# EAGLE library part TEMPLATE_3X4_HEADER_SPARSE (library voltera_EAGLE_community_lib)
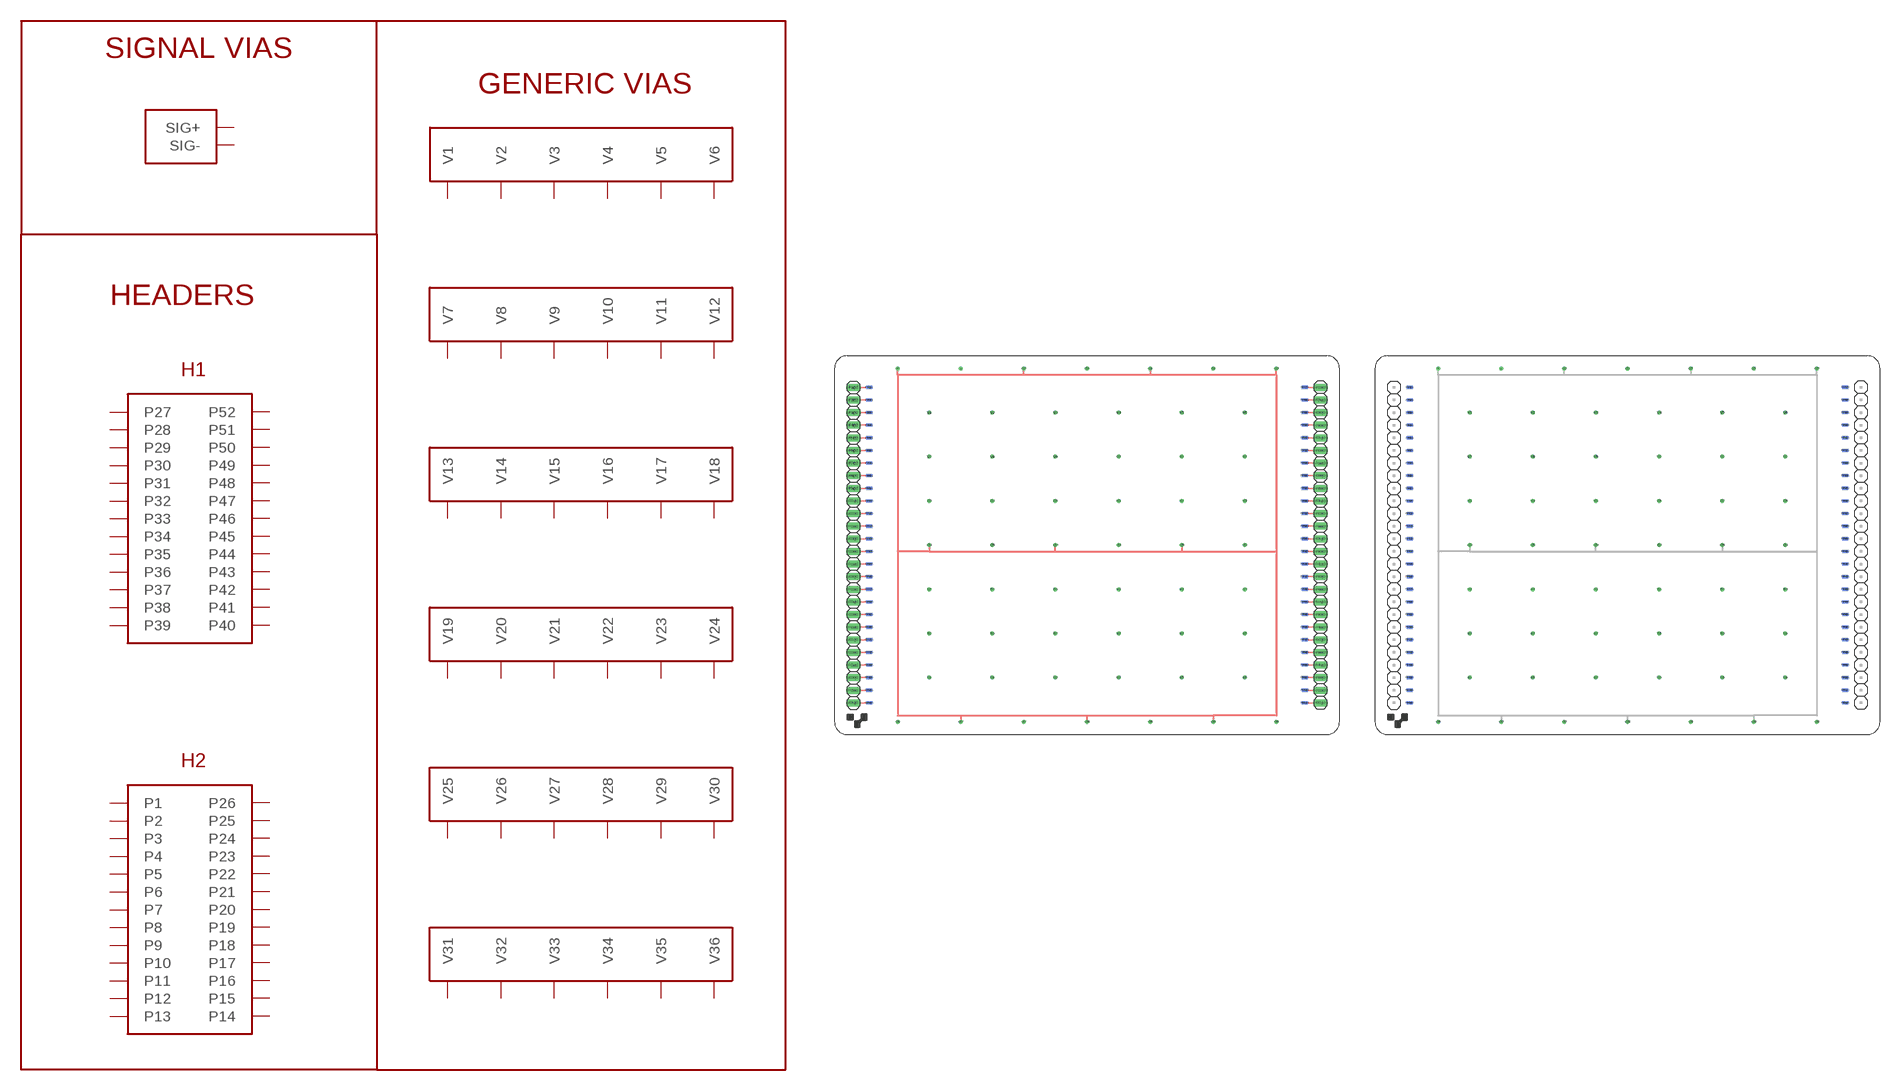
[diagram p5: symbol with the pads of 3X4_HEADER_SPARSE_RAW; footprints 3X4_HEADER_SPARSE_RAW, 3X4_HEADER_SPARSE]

Designator prefix -

## TEMPLATE_3X4_HEADER_SPARSE_RAW  [3X4_HEADER_SPARSE_RAW]
+  SIG+
+@1  SIG+
+@2  SIG+
+@3  SIG+
+@4  SIG+
+@5  SIG+
+@6  SIG+
+@7  SIG+
+@8  SIG+
+@9  SIG+
-  SIG-
-@1  SIG-
-@2  SIG-
-@3  SIG-
-@4  SIG-
-@5  SIG-
-@6  SIG-
-@7  SIG-
-@8  SIG-
-@9  SIG-
P1  P1
P1@1  P1
P1@2  P1
P2  P2
P2@1  P2
P2@2  P2
P3  P3
P3@1  P3
P3@2  P3
P4  P4
P4@1  P4
P4@2  P4
P5  P5
P5@1  P5
P5@2  P5
P6  P6
P6@1  P6
P6@2  P6
P7  P7
P7@1  P7
P7@2  P7
P8  P8
P8@1  P8
P8@2  P8
P9  P9
P9@1  P9
P9@2  P9
P10  P10
P10@1  P10
P10@2  P10
P11  P11
P11@1  P11
P11@2  P11
P12  P12
P12@1  P12
P12@2  P12
P13  P13
P13@1  P13
P13@2  P13
P14  P14
P14@1  P14
P14@2  P14
P15  P15
P15@1  P15
P15@2  P15
P16  P16
P16@1  P16
P16@2  P16
P17  P17
P17@1  P17
P17@2  P17
P18  P18
P18@1  P18
P18@2  P18
P19  P19
P19@1  P19
P19@2  P19
P20  P20
P20@1  P20
P20@2  P20
P21  P21
P21@1  P21
P21@2  P21
P22  P22
P22@1  P22
P22@2  P22
P23  P23
P23@1  P23
P23@2  P23
P24  P24
P24@1  P24
P24@2  P24
P25  P25
P25@1  P25
P25@2  P25
P26  P26
P26@1  P26
P26@2  P26
P27  P27
P27@1  P27
P27@2  P27
P28  P28
P28@1  P28
P28@2  P28
P29  P29
P29@1  P29
P29@2  P29
P30  P30
P30@1  P30
P30@2  P30
P31  P31
P31@1  P31
P31@2  P31
P32  P32
P32@1  P32
P32@2  P32
P33  P33
P33@1  P33
P33@2  P33
P34  P34
P34@1  P34
P34@2  P34
P35  P35
P35@1  P35
P35@2  P35
P36  P36
P36@1  P36
P36@2  P36
P37  P37
P37@1  P37
P37@2  P37
P38  P38
P38@1  P38
P38@2  P38
P39  P39
P39@1  P39
P39@2  P39
P40  P40
P40@1  P40
P40@2  P40
P41  P41
P41@1  P41
P41@2  P41
P42  P42
P42@1  P42
P42@2  P42
P43  P43
P43@1  P43
P43@2  P43
P44  P44
P44@1  P44
P44@2  P44
P45  P45
P45@1  P45
P45@2  P45
P46  P46
P46@1  P46
P46@2  P46
P47  P47
P47@1  P47
P47@2  P47
P48  P48
P48@1  P48
P48@2  P48
P49  P49
P49@1  P49
P49@2  P49
P50  P50
P50@1  P50
P50@2  P50
P51  P51
P51@1  P51
P51@2  P51
P52  P52
P52@1  P52
P52@2  P52
V1  V1
V2  V2
V3  V3
V4  V4
V5  V5
V6  V6
V7  V7
V8  V8
V9  V9
V10  V10
V11  V11
V12  V12
V13  V13
V14  V14
V15  V15
V16  V16
V17  V17
V18  V18
V19  V19
V20  V20
V21  V21
V22  V22
V23  V23
V24  V24
V25  V25
V26  V26
V27  V27
V28  V28
V29  V29
V30  V30
V31  V31
V32  V32
V33  V33
V34  V34
V35  V35
V36  V36

## TEMPLATE_3X4_HEADER_SPARSE_TEMPLATE  [3X4_HEADER_SPARSE]
+  SIG+
+@1  SIG+
+@2  SIG+
+@3  SIG+
+@4  SIG+
+@5  SIG+
+@6  SIG+
+@7  SIG+
+@8  SIG+
+@9  SIG+
-  SIG-
-@1  SIG-
-@2  SIG-
-@3  SIG-
-@4  SIG-
-@5  SIG-
-@6  SIG-
-@7  SIG-
-@8  SIG-
-@9  SIG-
P1  P1
P1@1  P1
P2  P2
P2@1  P2
P3  P3
P3@1  P3
P4  P4
P4@1  P4
P5  P5
P5@1  P5
P6  P6
P6@1  P6
P7  P7
P7@1  P7
P8  P8
P8@1  P8
P9  P9
P9@1  P9
P10  P10
P10@1  P10
P11  P11
P11@1  P11
P12  P12
P12@1  P12
P13  P13
P13@1  P13
P14  P14
P14@1  P14
P15  P15
P15@1  P15
P16  P16
P16@1  P16
P17  P17
P17@1  P17
P18  P18
P18@1  P18
P19  P19
P19@1  P19
P20  P20
P20@1  P20
P21  P21
P21@1  P21
P22  P22
P22@1  P22
P23  P23
P23@1  P23
P24  P24
P24@1  P24
P25  P25
P25@1  P25
P26  P26
P26@1  P26
P27  P27
P27@1  P27
P28  P28
P28@1  P28
P29  P29
P29@1  P29
P30  P30
P30@1  P30
P31  P31
P31@1  P31
P32  P32
P32@1  P32
P33  P33
P33@1  P33
P34  P34
P34@1  P34
P35  P35
P35@1  P35
P36  P36
P36@1  P36
P37  P37
P37@1  P37
P38  P38
P38@1  P38
P39  P39
P39@1  P39
P40  P40
P40@1  P40
P41  P41
P41@1  P41
P42  P42
P42@1  P42
P43  P43
P43@1  P43
P44  P44
P44@1  P44
P45  P45
P45@1  P45
P46  P46
P46@1  P46
P47  P47
P47@1  P47
P48  P48
P48@1  P48
P49  P49
P49@1  P49
P50  P50
P50@1  P50
P51  P51
P51@1  P51
P52  P52
P52@1  P52
V1  V1
V2  V2
V3  V3
V4  V4
V5  V5
V6  V6
V7  V7
V8  V8
V9  V9
V10  V10
V11  V11
V12  V12
V13  V13
V14  V14
V15  V15
V16  V16
V17  V17
V18  V18
V19  V19
V20  V20
V21  V21
V22  V22
V23  V23
V24  V24
V25  V25
V26  V26
V27  V27
V28  V28
V29  V29
V30  V30
V31  V31
V32  V32
V33  V33
V34  V34
V35  V35
V36  V36

## Footprint 3X4_HEADER_SPARSE_RAW (pad centres in mm)
drill 0.3 pad 0.8: + 12.7,73.66; +@1 38.1,73.66; +@2 63.5,73.66; +@3 19.05,38.1; +@4 44.45,38.1; +@5 69.85,38.1; +@6 88.9,73.66; +@7 25.4,2.54; +@8 50.8,2.54; +@9 76.2,2.54; - 25.4,73.66; -@1 50.8,73.66; -@2 76.2,73.66; -@3 82.55,38.1; -@4 57.15,38.1; -@5 31.75,38.1; -@6 12.7,2.54; -@7 38.1,2.54; -@8 63.5,2.54; -@9 88.9,2.54; V1 19.05,64.77; V2 31.75,64.77; V3 44.45,64.77; V4 57.15,64.77; V5 69.85,64.77; V6 82.55,64.77; V7 19.05,55.88; V8 31.75,55.88; V9 44.45,55.88; V10 57.15,55.88; V11 69.85,55.88; V12 82.55,55.88; V13 19.05,46.99; V14 31.75,46.99; V15 44.45,46.99; V16 57.15,46.99; V17 69.85,46.99; V18 82.55,46.99; V19 19.05,29.21; V20 31.75,29.21; V21 44.45,29.21; V22 57.15,29.21; V23 69.85,29.21; V24 82.55,29.21; V25 19.05,20.32; V26 31.75,20.32; V27 44.45,20.32; V28 57.15,20.32; V29 69.85,20.32; V30 82.55,20.32; V31 19.05,11.43; V32 31.75,11.43; V33 44.45,11.43; V34 57.15,11.43; V35 69.85,11.43; V36 82.55,11.43
smd 1.27 x 0.635: P1 6.985,69.85; P2 6.985,67.31; P3 6.985,64.77; P4 6.985,62.23; P5 6.985,59.69; P6 6.985,57.15; P7 6.985,54.61; P8 6.985,52.07; P9 6.985,49.53; P10 6.985,46.99; P11 6.985,44.45; P12 6.985,41.91; P13 6.985,39.37; P14 6.985,36.83; P15 6.985,34.29; P16 6.985,31.75; P17 6.985,29.21; P18 6.985,26.67; P19 6.985,24.13; P20 6.985,21.59; P21 6.985,19.05; P22 6.985,16.51; P23 6.985,13.97; P24 6.985,11.43; P25 6.985,8.89; P26 6.985,6.35; P27 94.615,69.85; P28 94.615,67.31; P29 94.615,64.77; P30 94.615,62.23; P31 94.615,59.69; P32 94.615,57.15; P33 94.615,54.61; P34 94.615,52.07; P35 94.615,49.53; P36 94.615,46.99; P37 94.615,44.45; P38 94.615,41.91; P39 94.615,39.37; P40 94.615,36.83; P41 94.615,34.29; P42 94.615,31.75; P43 94.615,29.21; P44 94.615,26.67; P45 94.615,24.13; P46 94.615,21.59; P47 94.615,19.05; P48 94.615,16.51; P49 94.615,13.97; P50 94.615,11.43; P51 94.615,8.89; P52 94.615,6.35
smd 1.27 x 0.635 bottom: P1@1 6.985,69.85; P2@1 6.985,67.31; P3@1 6.985,64.77; P4@1 6.985,62.23; P5@1 6.985,59.69; P6@1 6.985,57.15; P7@1 6.985,54.61; P8@1 6.985,52.07; P9@1 6.985,49.53; P10@1 6.985,46.99; P11@1 6.985,44.45; P12@1 6.985,41.91; P13@1 6.985,39.37; P14@1 6.985,36.83; P15@1 6.985,34.29; P16@1 6.985,31.75; P17@1 6.985,29.21; P18@1 6.985,26.67; P19@1 6.985,24.13; P20@1 6.985,21.59; P21@1 6.985,19.05; P22@1 6.985,16.51; P23@1 6.985,13.97; P24@1 6.985,11.43; P25@1 6.985,8.89; P26@1 6.985,6.35; P27@1 94.615,69.85; P28@1 94.615,67.31; P29@1 94.615,64.77; P30@1 94.615,62.23; P31@1 94.615,59.69; P32@1 94.615,57.15; P33@1 94.615,54.61; P34@1 94.615,52.07; P35@1 94.615,49.53; P36@1 94.615,46.99; P37@1 94.615,44.45; P38@1 94.615,41.91; P39@1 94.615,39.37; P40@1 94.615,36.83; P41@1 94.615,34.29; P42@1 94.615,31.75; P43@1 94.615,29.21; P44@1 94.615,26.67; P45@1 94.615,24.13; P46@1 94.615,21.59; P47@1 94.615,19.05; P48@1 94.615,16.51; P49@1 94.615,13.97; P50@1 94.615,11.43; P51@1 94.615,8.89; P52@1 94.615,6.35
drill 1.016 long: P1@2 3.81,69.85; P2@2 3.81,67.31; P3@2 3.81,64.77; P4@2 3.81,62.23; P5@2 3.81,59.69; P6@2 3.81,57.15; P7@2 3.81,54.61; P8@2 3.81,52.07; P9@2 3.81,49.53; P10@2 3.81,46.99; P11@2 3.81,44.45; P12@2 3.81,41.91; P13@2 3.81,39.37; P14@2 3.81,36.83; P15@2 3.81,34.29; P16@2 3.81,31.75; P17@2 3.81,29.21; P18@2 3.81,26.67; P19@2 3.81,24.13; P20@2 3.81,21.59; P21@2 3.81,19.05; P22@2 3.81,16.51; P23@2 3.81,13.97; P24@2 3.81,11.43; P25@2 3.81,8.89; P26@2 3.81,6.35; P27@2 97.79,69.85; P28@2 97.79,67.31; P29@2 97.79,64.77; P30@2 97.79,62.23; P31@2 97.79,59.69; P32@2 97.79,57.15; P33@2 97.79,54.61; P34@2 97.79,52.07; P35@2 97.79,49.53; P36@2 97.79,46.99; P37@2 97.79,44.45; P38@2 97.79,41.91; P39@2 97.79,39.37; P40@2 97.79,36.83; P41@2 97.79,34.29; P42@2 97.79,31.75; P43@2 97.79,29.21; P44@2 97.79,26.67; P45@2 97.79,24.13; P46@2 97.79,21.59; P47@2 97.79,19.05; P48@2 97.79,16.51; P49@2 97.79,13.97; P50@2 97.79,11.43; P51@2 97.79,8.89; P52@2 97.79,6.35

## Footprint 3X4_HEADER_SPARSE (pad centres in mm)
drill 0.3 pad 0.8: + 12.7,73.66; +@1 38.1,73.66; +@2 63.5,73.66; +@3 19.05,38.1; +@4 44.45,38.1; +@5 69.85,38.1; +@6 88.9,73.66; +@7 25.4,2.54; +@8 50.8,2.54; +@9 76.2,2.54; - 25.4,73.66; -@1 50.8,73.66; -@2 76.2,73.66; -@3 82.55,38.1; -@4 57.15,38.1; -@5 31.75,38.1; -@6 12.7,2.54; -@7 38.1,2.54; -@8 63.5,2.54; -@9 88.9,2.54; V1 19.05,64.77; V2 31.75,64.77; V3 44.45,64.77; V4 57.15,64.77; V5 69.85,64.77; V6 82.55,64.77; V7 19.05,55.88; V8 31.75,55.88; V9 44.45,55.88; V10 57.15,55.88; V11 69.85,55.88; V12 82.55,55.88; V13 19.05,46.99; V14 31.75,46.99; V15 44.45,46.99; V16 57.15,46.99; V17 69.85,46.99; V18 82.55,46.99; V19 19.05,29.21; V20 31.75,29.21; V21 44.45,29.21; V22 57.15,29.21; V23 69.85,29.21; V24 82.55,29.21; V25 19.05,20.32; V26 31.75,20.32; V27 44.45,20.32; V28 57.15,20.32; V29 69.85,20.32; V30 82.55,20.32; V31 19.05,11.43; V32 31.75,11.43; V33 44.45,11.43; V34 57.15,11.43; V35 69.85,11.43; V36 82.55,11.43
smd 1.27 x 0.635: P1 6.985,69.85; P2 6.985,67.31; P3 6.985,64.77; P4 6.985,62.23; P5 6.985,59.69; P6 6.985,57.15; P7 6.985,54.61; P8 6.985,52.07; P9 6.985,49.53; P10 6.985,46.99; P11 6.985,44.45; P12 6.985,41.91; P13 6.985,39.37; P14 6.985,36.83; P15 6.985,34.29; P16 6.985,31.75; P17 6.985,29.21; P18 6.985,26.67; P19 6.985,24.13; P20 6.985,21.59; P21 6.985,19.05; P22 6.985,16.51; P23 6.985,13.97; P24 6.985,11.43; P25 6.985,8.89; P26 6.985,6.35; P27 94.615,69.85; P28 94.615,67.31; P29 94.615,64.77; P30 94.615,62.23; P31 94.615,59.69; P32 94.615,57.15; P33 94.615,54.61; P34 94.615,52.07; P35 94.615,49.53; P36 94.615,46.99; P37 94.615,44.45; P38 94.615,41.91; P39 94.615,39.37; P40 94.615,36.83; P41 94.615,34.29; P42 94.615,31.75; P43 94.615,29.21; P44 94.615,26.67; P45 94.615,24.13; P46 94.615,21.59; P47 94.615,19.05; P48 94.615,16.51; P49 94.615,13.97; P50 94.615,11.43; P51 94.615,8.89; P52 94.615,6.35
smd 1.27 x 0.635 bottom: P1@1 6.985,69.85; P2@1 6.985,67.31; P3@1 6.985,64.77; P4@1 6.985,62.23; P5@1 6.985,59.69; P6@1 6.985,57.15; P7@1 6.985,54.61; P8@1 6.985,52.07; P9@1 6.985,49.53; P10@1 6.985,46.99; P11@1 6.985,44.45; P12@1 6.985,41.91; P13@1 6.985,39.37; P14@1 6.985,36.83; P15@1 6.985,34.29; P16@1 6.985,31.75; P17@1 6.985,29.21; P18@1 6.985,26.67; P19@1 6.985,24.13; P20@1 6.985,21.59; P21@1 6.985,19.05; P22@1 6.985,16.51; P23@1 6.985,13.97; P24@1 6.985,11.43; P25@1 6.985,8.89; P26@1 6.985,6.35; P27@1 94.615,69.85; P28@1 94.615,67.31; P29@1 94.615,64.77; P30@1 94.615,62.23; P31@1 94.615,59.69; P32@1 94.615,57.15; P33@1 94.615,54.61; P34@1 94.615,52.07; P35@1 94.615,49.53; P36@1 94.615,46.99; P37@1 94.615,44.45; P38@1 94.615,41.91; P39@1 94.615,39.37; P40@1 94.615,36.83; P41@1 94.615,34.29; P42@1 94.615,31.75; P43@1 94.615,29.21; P44@1 94.615,26.67; P45@1 94.615,24.13; P46@1 94.615,21.59; P47@1 94.615,19.05; P48@1 94.615,16.51; P49@1 94.615,13.97; P50@1 94.615,11.43; P51@1 94.615,8.89; P52@1 94.615,6.35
